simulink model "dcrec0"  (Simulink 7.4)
settings: Solver=ode45  StartTime=0.0  StopTime=0.01  MaxStep=1e-4  RelTol=1e-3

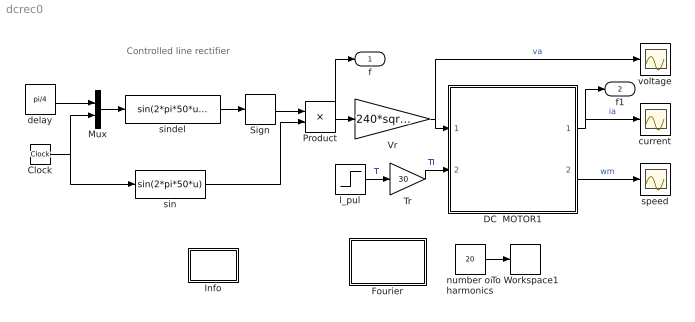
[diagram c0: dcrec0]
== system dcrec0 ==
  note: Controlled line rectifier
  Clock : Clock
  DC  MOTOR1 : Subsystem  mask{Ra=0.60, La=0.1, J=0.6, Bm=1e-5, K=1.85}
      mask prompts: Ra "Armature resistance [ohm]"; La "Armature inductance [H]"; J "Moment of inertia [Kg.m^2]"; Bm "Frictional torque cefficient"; K "Electromechanical coupling coefficient [N.m/A]"
  Fourier : Subsystem
  Info : Subsystem
  Mux : Mux  Inputs=2
  Product : Product  OutDataType=sfix(16)  OutScaling=2^0
  Sign : Signum
  To Workspace1 : ToWorkspace  VariableName=h  SampleTime=-1  SaveFormat=Array
  Tr : Gain  Gain=30  ParameterDataType=sfix(16)  ParameterScaling=2^0  OutDataType=sfix(16)  OutScaling=2^0
  Vr : Gain  Gain=240*sqrt(2)  ParameterDataType=sfix(16)  ParameterScaling=2^0  OutDataType=sfix(16)  OutScaling=2^0
  current : Scope
  delay : Constant  Value=pi/4  OutDataType=sfix(16)  OutScaling=2^0
  l_pul : Step  Time=0.1  Before=1  SampleTime=0
  number of harmonics : Constant  Value=20  OutDataType=sfix(16)  OutScaling=2^0
  sin : Fcn  Expr=sin(2*pi*50*u)
  sindel : Fcn  Expr=sin(2*pi*50*u(2)-u(1))
  speed : Scope
  voltage : Scope
  f : Outport
  f1 : Outport  Port=2
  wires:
  Sign/1 -> Product/1
  sindel/1 -> Sign/1
  sin/1 -> Product/2
  Mux/1 -> sindel/1
  Clock/1 -> Mux/2, sin/1
  delay/1 -> Mux/1
  Vr/1 -> voltage/1, DC  MOTOR1/1(va)  "va"
  l_pul/1 -> Tr/1  "Tl"
  Product/1 -> Vr/1, f/1
  DC  MOTOR1/2(wm) -> speed/1  "wm"
  number of harmonics/1 -> To Workspace1/1
  DC  MOTOR1/1(ia) -> current/1, f1/1  "ia"
  Tr/1 -> DC  MOTOR1/2(Tl)  "Tl"

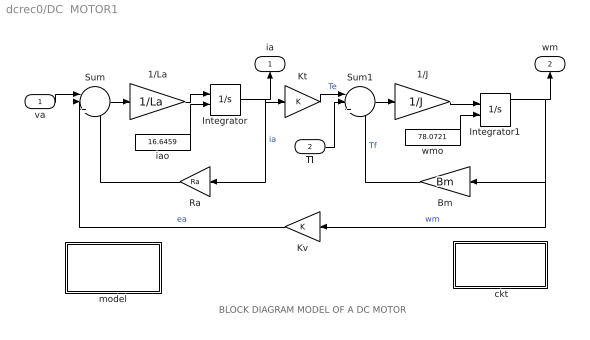
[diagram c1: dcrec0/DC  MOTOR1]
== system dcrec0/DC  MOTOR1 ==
  note: BLOCK DIAGRAM MODEL OF A DC MOTOR
  va : Inport  OutDataType=sfix(16)  OutScaling=2^0
  Tl : Inport  Port=2  OutDataType=sfix(16)  OutScaling=2^0
  " ckt" : Subsystem
  1/J : Gain  Gain=1/J  ParameterDataType=sfix(16)  ParameterScaling=2^0  OutDataType=sfix(16)  OutScaling=2^0
  1/La : Gain  Gain=1/La  ParameterDataType=sfix(16)  ParameterScaling=2^0  OutDataType=sfix(16)  OutScaling=2^0
  Bm : Gain  Gain=Bm  ParameterDataType=sfix(16)  ParameterScaling=2^0  OutDataType=sfix(16)  OutScaling=2^0
  Integrator : Integrator  InitialConditionSource=external  InitialCondition=16.2162
  Integrator1 : Integrator  InitialConditionSource=external  InitialCondition=98.5245
  Kt : Gain  Gain=K  ParameterDataType=sfix(16)  ParameterScaling=2^0  OutDataType=sfix(16)  OutScaling=2^0
  Kv : Gain  Gain=K  ParameterDataType=sfix(16)  ParameterScaling=2^0  OutDataType=sfix(16)  OutScaling=2^0
  Ra : Gain  Gain=Ra  ParameterDataType=sfix(16)  ParameterScaling=2^0  OutDataType=sfix(16)  OutScaling=2^0
  Sum : Sum  Inputs=||+--  OutDataType=sfix(16)  OutScaling=2^0
  Sum1 : Sum  Inputs=||+--  OutDataType=sfix(16)  OutScaling=2^0
  iao : Constant  Value=16.6459  OutDataType=sfix(16)  OutScaling=2^0
  model : Subsystem
  wmo : Constant  Value=78.0721  OutDataType=sfix(16)  OutScaling=2^0
  ia : Outport
  wm : Outport  Port=2
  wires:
  Kv/1 -> Sum/2  "ea"
  Ra/1 -> Sum/3
  Kt/1 -> Sum1/1  "Te"
  Bm/1 -> Sum1/3  "Tf"
  Sum/1 -> 1/La/1
  1/La/1 -> Integrator/1
  Integrator/1 -> Ra/1, Kt/1, ia/1  "ia"
  Sum1/1 -> 1/J/1
  1/J/1 -> Integrator1/1
  Integrator1/1 -> Bm/1, Kv/1, wm/1  "wm"
  va/1 -> Sum/1
  Tl/1 -> Sum1/2
  iao/1 -> Integrator/2
  wmo/1 -> Integrator1/2

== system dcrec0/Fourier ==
  note: To obtain the Fourier decomposition of a periodic signal: a) run a simulation for one period duration b) Specify the fundamental frequency c) Specify the number of harmonics

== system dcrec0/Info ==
  note: This demo simulates the running of a DC motor with controlled (thyristor) line rectification (5 hp 240V 1200 rpm) rated torque Tr = 30 N.m]

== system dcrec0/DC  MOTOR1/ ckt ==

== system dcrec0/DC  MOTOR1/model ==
  note: Electrical system equation: va = Ra.ia + La.dia/dt + ea where ea = K.wm Mechanical system equation: Te = J.dwm/dt + Tl.signum(wm) + f(wm) where Te = K.ia
  note: Mathematical model of the dc machine
